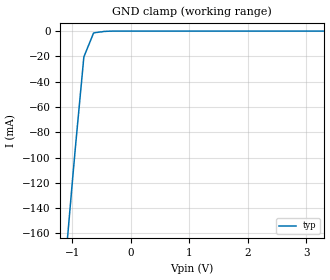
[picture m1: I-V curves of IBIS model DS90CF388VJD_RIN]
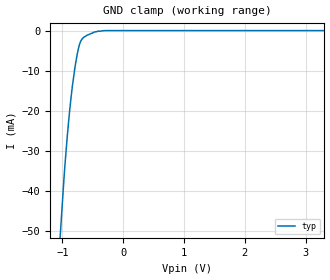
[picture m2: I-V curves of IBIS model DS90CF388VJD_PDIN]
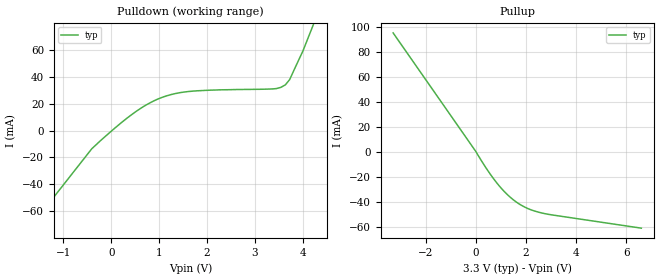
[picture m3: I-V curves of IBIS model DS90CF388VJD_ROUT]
|   National Semiconductor Corporation
|   Interface Products Group
|   IBIS Model of Channel Link Receiver
|   100VJD TQFP
[IBIS Ver]   2.1
[Comment char]  |_char
[File name]   cf388vjd.ibs
[File Rev]   2.1
[Date]   8/29/2001
[Source]   File originated at National Semiconductor Corporation.
   Interface Group/Analog Division. All data based on
   Empirical Measurements(Bench).
[Notes]   File created by CW.
   Revision 1: The original model
   Revision 2: Change "vdiff" values from "NA" to 0.1
   Revision 2.1: redo RIN GND_clamp data, bad values
   around 0 volts---milt
[Disclaimer]
(C) Copyright National Semiconductor Corporation 1999
   All rights reserved
   National Semiconductor Corporation hereby grants
the user of this IBIS model a non-exclusive, nontransferable
license to use this IBIS model under the following terms.
Before using this IBIS model, the user should read this
license.  If the user does not accept these terms,  the
IBIS model should be returned to National within 30 days.
   The user is granted this license only to use the
IBIS model and is not granted rights to sell, load, rent,
lease or license the IBIS model in whole or in part, or in
modified form to anyone other than user. User may modify
the IBIS model to suit its specific applications but rights
to derivative works and such modifications shall belong to
National.
   This IBIS model is provided on an "AS IS" basis and
National makes absolutely no warranty with respect to the
information contained herein.NATIONAL DISCLAIMS AND CUSTOMER
WAIVES ALL WARRANTIES, EXPRESS OR IMPLIED, INCLUDING
WARRANTIES OF MERCHANTABILITY OR FITNESS FOR A PARTICULAR
PURPOSE. The entire risk as to quality and performance is
with the Customer. ACCORDINGLY, IN NO EVENT SHALL THE
COMPANY BE LIABLE FOR ANY DAMAGES, WHETHER IN CONTRACT OR
TORT,INCLUDING ANY LOST PROFITS OR OTHER INCIDENTAL,
CONSEQUENTIAL, EXEMPLARY, OR PUNITIVE DAMAGES ARISING OUT
OF THE USE OR APPLICATION OF THE IBIS model provided in
this package.Further, National reserves the right to make
changes without notice to any product herein to improve
reliability, function, or design. National does not convey
any license under patent rights or any other intellectual
property rights, including those of third parties.
   National is not obligated to provide maintenance or support
for the licensed IBIS model.
Contact National at ATTN:INTERFACE APPLICATIONS/IBIS MODELS.
2900 Semiconductor Drive, M/S A2595, Santa Clara, CA 95052-8090
[Copyright]   Copyright 1999, National Semiconductor, All Rights Reserved
[Component]   DS90CF388VJD
[Manufacturer]  National Semiconductor Corp
[Package]
|   typ   min   max
R_pkg   64.20m   NA   NA
L_pkg   2.491nH   NA   NA
C_pkg   0.3380pF   NA   NA
[Pin]   signal_name   model_name   R_pin   L_pin   C_pin
1   PLLGND   GND   70.72m  2.917n   0.3789p
2   PLLVCC   POWER   70.51m  2.771n   0.3776p
3   PLLGND   GND   68.62m  2.713n   0.3658p
4   DESKEW   DS90CF388VJD_PDIN   67.20m  2.650n   0.3568p
5   PLLSEL   DS90CF388VJD_PDIN   65.58m  2.545n   0.3467p
6   BAL   DS90CF388VJD_PDIN   64.85m  2.496n   0.3421p
7   GND   GND   63.40m  2.419n   0.3328p
8   RxOUTR10   DS90CF388VJD_ROUT   62.50m  2.437n   0.3272p
9   RxOUTR11   DS90CF388VJD_ROUT   61.19m  2.376n   0.3192p
10   RxOUTR12   DS90CF388VJD_ROUT   60.16m  2.276n   0.3127p
11   RxOUTR13   DS90CF388VJD_ROUT   59.45m  2.239n   0.3083p
12   RxOUTR14   DS90CF388VJD_ROUT   58.73m  2.205n   0.3038p
13   VCC   POWER   59.19m  2.179n   0.3067p
14   RxOUTR15   DS90CF388VJD_ROUT   58.73m  2.205n   0.3038p
15   RxOUTR16   DS90CF388VJD_ROUT   59.45m  2.239n   0.3083p
16   GND   GND   60.16m  2.276n   0.3127p
17   RxOUTR17   DS90CF388VJD_ROUT   61.19m  2.376n   0.3192p
18   RxOUTG10   DS90CF388VJD_ROUT   62.50m  2.437n   0.3272p
19   RxOUTG11   DS90CF388VJD_ROUT   63.40m  2.419n   0.3328p
20   RxOUTG12   DS90CF388VJD_ROUT   64.85m  2.496n   0.3421p
21   RxOUTG13   DS90CF388VJD_ROUT   65.58m  2.545n   0.3467p
22   RxOUTG14   DS90CF388VJD_ROUT   67.20m  2.650n   0.3568p
23   VCC   POWER   68.62m  2.713n   0.3658p
24   RxOUTG15   DS90CF388VJD_ROUT   70.51m  2.771n   0.3776p
25   GND   GND   70.72m  2.917n   0.3789p
26   RxOUTG16   DS90CF388VJD_ROUT   70.72m  2.917n   0.3789p
27   RxOUTG17   DS90CF388VJD_ROUT   70.51m  2.771n   0.3776p
28   RxOUTB10   DS90CF388VJD_ROUT   68.62m  2.713n   0.3658p
29   RxOUTB11   DS90CF388VJD_ROUT   67.20m  2.650n   0.3568p
30   RxOUTB12   DS90CF388VJD_ROUT   65.58m  2.545n   0.3467p
31   RxOUTB13   DS90CF388VJD_ROUT   64.85m  2.496n   0.3421p
32   RxOUTB14   DS90CF388VJD_ROUT   63.40m  2.419n   0.3328p
33   VCC   POWER   62.50m  2.437n   0.3272p
34   RxOUTB15   DS90CF388VJD_ROUT   61.19m  2.376n   0.3192p
35   GND   GND   60.16m  2.276n   0.3127p
36   RxOUTB16   DS90CF388VJD_ROUT   59.45m  2.239n   0.3083p
37   RxOUTB17   DS90CF388VJD_ROUT   58.73m  2.205n   0.3038p
38   RxOUTR20   DS90CF388VJD_ROUT   59.19m  2.179n   0.3067p
39   RxOUTR21   DS90CF388VJD_ROUT   58.73m  2.205n   0.3038p
40   RxOUTR22   DS90CF388VJD_ROUT   59.45m  2.239n   0.3083p
41   RxOUTR23   DS90CF388VJD_ROUT   60.16m  2.276n   0.3127p
42   CLKOUT   DS90CF388VJD_ROUT   61.19m  2.376n   0.3192p
43   RxOUTR24   DS90CF388VJD_ROUT   62.50m  2.437n   0.3272p
44   GND   GND   63.40m  2.419n   0.3328p
45   VCC   POWER   64.85m  2.496n   0.3421p
46   RxOUTR25   DS90CF388VJD_ROUT   65.58m  2.545n   0.3467p
47   RxOUTR26   DS90CF388VJD_ROUT   67.20m  2.650n   0.3568p
48   RxOUTR27   DS90CF388VJD_ROUT   68.62m  2.713n   0.3658p
49   RxOUTG20   DS90CF388VJD_ROUT   70.51m  2.771n   0.3776p
50   RxOUTG21   DS90CF388VJD_ROUT   70.72m  2.917n   0.3789p
51   RxOUTG22   DS90CF388VJD_ROUT   70.72m  2.917n   0.3789p
52   RxOUTG23   DS90CF388VJD_ROUT   70.51m  2.771n   0.3776p
53   RxOUTG24   DS90CF388VJD_ROUT   68.62m  2.713n   0.3658p
54   GND   GND   67.20m  2.650n   0.3568p
55   RxOUTG25   DS90CF388VJD_ROUT   65.58m  2.545n   0.3467p
56   VCC   POWER   64.85m  2.496n   0.3421p
57   RxOUTG26   DS90CF388VJD_ROUT   63.40m  2.419n   0.3328p
58   RxOUTG27   DS90CF388VJD_ROUT   62.50m  2.437n   0.3272p
59   RxOUTB20   DS90CF388VJD_ROUT   61.19m  2.376n   0.3192p
60   RxOUTB21   DS90CF388VJD_ROUT   60.16m  2.276n   0.3127p
61   RxOUTB22   DS90CF388VJD_ROUT   59.45m  2.239n   0.3083p
62   RxOUTB23   DS90CF388VJD_ROUT   58.73m  2.205n   0.3038p
63   GND   GND   59.19m  2.179n   0.3067p
64   RxOUTB24   DS90CF388VJD_ROUT   58.73m  2.205n   0.3038p
65   RxOUTB25   DS90CF388VJD_ROUT   59.45m  2.239n   0.3083p
66   VCC   POWER   60.16m  2.276n   0.3127p
67   RxOUTB26   DS90CF388VJD_ROUT   61.19m  2.376n   0.3192p
68   RxOUTB27   DS90CF388VJD_ROUT   62.50m  2.437n   0.3272p
69   DE   DS90CF388VJD_ROUT   63.40m  2.419n   0.3328p
70   VSYNC   DS90CF388VJD_ROUT   64.85m  2.496n   0.3421p
71   HSYNC   DS90CF388VJD_ROUT   65.58m  2.545n   0.3467p
72   GND   GND   67.20m  2.650n   0.3568p
73   STOPCLK   DS90CF388VJD_ROUT   68.62m  2.713n   0.3658p
74   CNTLF   DS90CF388VJD_ROUT   70.51m  2.771n   0.3776p
75   CNTLE   DS90CF388VJD_ROUT   70.72m  2.917n   0.3789p
76   LVDSGND   GND   70.72m  2.917n   0.3789p
77   RF_DE   DS90CF388VJD_PDIN   70.51m  2.771n   0.3776p
78   PD*   DS90CF388VJD_PDIN   68.62m  2.713n   0.3658p
79   A7P   DS90CF388VJD_RIN   67.20m  2.650n   0.3568p
80   A7M   DS90CF388VJD_RIN   65.58m  2.545n   0.3467p
81   LVDSVCC   POWER   64.85m  2.496n   0.3421p
82   A6P   DS90CF388VJD_RIN   63.40m  2.419n   0.3328p
83   A6M   DS90CF388VJD_RIN   62.50m  2.437n   0.3272p
84   A5P   DS90CF388VJD_RIN   61.19m  2.376n   0.3192p
85   A5M   DS90CF388VJD_RIN   60.16m  2.276n   0.3127p
86   A4P   DS90CF388VJD_RIN   59.45m  2.239n   0.3083p
87   A4M   DS90CF388VJD_RIN   58.73m  2.205n   0.3038p
88   LVDSGND   GND   59.19m  2.179n   0.3067p
89   A3P   DS90CF388VJD_RIN   58.73m  2.205n   0.3038p
90   A3M   DS90CF388VJD_RIN   59.45m  2.239n   0.3083p
91   CLKP   DS90CF388VJD_RIN   60.16m  2.276n   0.3127p
92   CLKM   DS90CF388VJD_RIN   61.19m  2.376n   0.3192p
93   LVDSVCC   POWER   62.50m  2.437n   0.3272p
94   A2P   DS90CF388VJD_RIN   63.40m  2.419n   0.3328p
95   A2M   DS90CF388VJD_RIN   64.85m  2.496n   0.3421p
96   A1P   DS90CF388VJD_RIN   65.58m  2.545n   0.3467p
97   A1M   DS90CF388VJD_RIN   67.20m  2.650n   0.3568p
98   A0P   DS90CF388VJD_RIN   68.62m  2.713n   0.3658p
99   A0M   DS90CF388VJD_RIN   70.51m  2.771n   0.3776p
100   LVDSGND   GND   70.72m  2.917n   0.3789p
[Diff_pin]   inv_pin   vdiff   tdelay_typ   tdelay_min   tdelay_max
| The '+' pin is Diff_pin and the '-' pin is the inv_pin
79   80   0.1   0   0   0
82   83   0.1   0   0   0
84   85   0.1   0   0   0
86   87   0.1   0   0   0
89   90   0.1   0   0   0
91   92   0.1   0   0   0
94   95   0.1   0   0   0
96   97   0.1   0   0   0
98   99   0.1   0   0   0
| Models and submodels in the file (3): DS90CF388VJD_RIN (Input), DS90CF388VJD_PDIN (Input), DS90CF388VJD_ROUT (3-state)
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|   RECEIVER INPUT MODEL
[Model]   DS90CF388VJD_RIN
Model_type   Input
|Signals   A0M ~ A7M, A0P ~ A7P, CLKP, CLKM
Vinh = 2.0
Vinl = 0.8
|   typ   min   max
C_comp   5.830pF   NA   NA
|   typ   min   max
[Temperature Range]   25.0   NA   NA
[Voltage range]   3.3V   3.0V   3.6V
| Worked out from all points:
|   GND clamp passes 1 mA (typ) near -0.57 V on its own axis
[Power_clamp]
| Note that the [POWER_clamp] voltage table is referenced to Vcc
| and is calculated using Vtable = Vcc - Vmeasured.
|Voltage   I(typ)   I(min)   I(max)
-3V       0A         NA         NA
0V        0A         NA         NA
[GND_clamp]
|Voltage   I(typ)   I(min)  I(max)
-3.3V     -1.356A    NA         NA
-1V       -121mA     NA         NA
-943mV    -91.17mA   NA         NA
-800mV    -20.46mA   NA         NA
-633.9mV  -1.52mA    NA         NA
-285.7mV  -7.86uA    NA         NA
3.3V      -50.7nA    NA         NA
|   RECEIVER PWRDWN* INPUT MODEL
[Model]   DS90CF388VJD_PDIN
Model_type   Input
|Signals   PD*, PLLSEL, DESKEW, RF_DE, BAL
Vinh = 2.0
Vinl = 0.8
|   typ   min   max
C_comp   5.832pF   NA   NA
|   typ   min   max
[Temperature Range]   25.0   NA   NA
[Voltage range]   3.3V   3.0V   3.6V
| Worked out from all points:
|   GND clamp passes 1 mA (typ) near -0.57 V on its own axis
[Power_clamp]
| Note that the [POWER_clamp] voltage table is referenced to Vcc
| and is calculated using Vtable = Vcc - Vmeasured.
|Voltage   I(typ)   I(min)   I(max)
-3.3V     0A         0A         0A
0V        0A         0A         0A
[GND_clamp]
|Voltage   I(typ)   I(min)   I(max)
-3.3V     -576.3mA   NA         NA
-1.001V   -42.99mA   NA         NA
-961.4mV  -34.06mA   NA         NA
-898.9mV  -22.73mA   NA         NA
-858.1mV  -16.66mA   NA         NA
-797.1mV  -9.469mA   NA         NA
-756.3mV  -5.884mA   NA         NA
-714.5mV  -3.211mA   NA         NA
-654mV    -1.71mA    NA         NA
-592.6mV  -1.13mA    NA         NA
-285.7mV  -7.858uA   NA         NA
3.3V      -50.7nA    NA         NA
|   RECEIVER OUTPUT MODEL
[Model]   DS90CF388VJD_ROUT
Model_type   3-state
|Signals   RxOUTR10 ~ RxOUTR17, RxOUTR20 ~ RxOUTR27, RxOUTG10 ~ RxOUTG17,
|   RxOUTG20 ~ RxOUTG27, RxOUTB10 ~ RxOUTB17, RxOUTB20 ~ RxOUTB27,
|   DE, HSYNC, VSYNC, CNTLE, CNTLF, STOPCLK, CLKOUT
Vmeas = 1.5V   |This is 0.0v differential on ouput
Cref = 8pF   |Timing specification test load capacitance value
Vref = 0   |Timing specification test load voltage; GND
|variable   typ   min   max
C_comp   6.070pF   NA   NA
|   typ   min   max
[Temperature Range]   25.0   NA   NA
[Voltage range]   3.3V   3.0V   3.6V
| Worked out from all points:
|   slope of the pulldown table from 0 to 0.495 V, typ, clamps not added: 35.2 ohm
|   slope of the pullup table from 0 to 0.495 V, typ, clamps not added: 31.4 ohm
[Pulldown]
|Voltage   I(typ)   I(min)   I(max)
-3.3V     -144.4mA   NA         NA
-500.6mV  -17.74mA   NA         NA
-226.2mV  -7.519mA   NA         NA
326.5mV   9.15mA     NA         NA
969.7mV   23.34mA    NA         NA
1.612V    28.96mA    NA         NA
3.541V    32.06mA    NA         NA
3.632V    33.85mA    NA         NA
3.724V    37.86mA    NA         NA
3.999V    58.96mA    NA         NA
4.5V      103.9mA    NA         NA
6.6V      337.2mA    NA         NA
[Pullup]
| Note that the [Pullup] voltage table is referenced to Vcc
| and is calculated using Vtable = Vcc - Vmeasured.
|Voltage   I(typ)   I(min)   I(max)
-3.3V     95.33mA    NA         NA
-167.1uV  457.9uA    NA         NA
336.7mV   -10.55mA   NA         NA
607.2mV   -18.54mA   NA         NA
1.01V     -28.84mA   NA         NA
1.482V    -37.96mA   NA         NA
1.751V    -41.75mA   NA         NA
2.087V    -45.26mA   NA         NA
2.694V    -48.96mA   NA         NA
6.6V      -60.83mA   NA         NA
[GND_clamp]
| Outputs in Tri-state.
|Voltage   I(typ)   I(min)   I(max)
| Receiver output is non-tristable
-3V       0A         NA         NA
3V        0A         NA         NA
[POWER_clamp]
| Note that the [POWER_clamp] voltage table is referenced to Vcc
| and is calculated using Vtable = Vcc - Vmeasured.
| Outputs in Tri-state.
|Voltage   I(typ)   I(min)   I(max)
| Receiver output is non-tristable
-3V       0A         NA         NA
0V        0A         NA         NA
[Ramp]
|   typ   min   max
dV/dt_r   1.98/1.520n   NA   NA
dV/dt_f   1.98/1.700n   NA   NA
R_load = 1MOhm  | Represent Hi-Z
